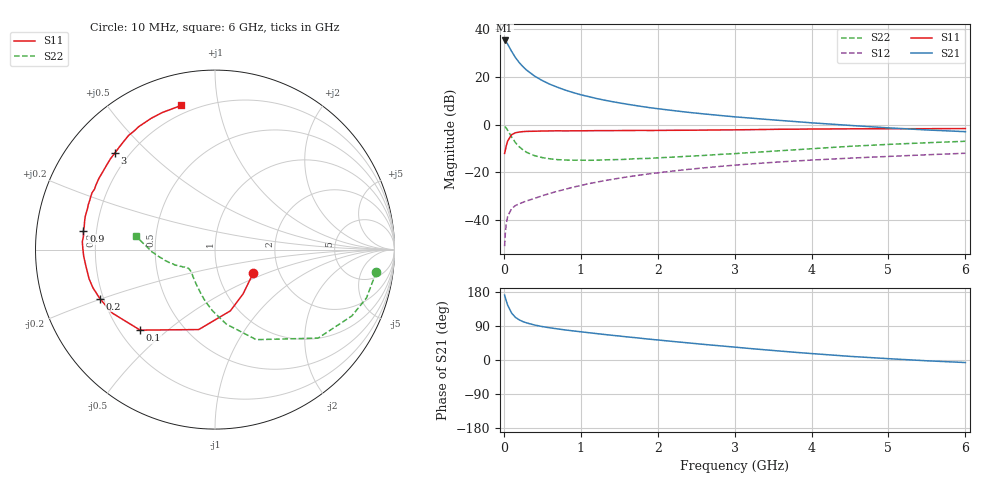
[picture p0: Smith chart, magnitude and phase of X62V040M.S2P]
! SIEMENS Small Signal Semiconductors
! BFP193W
! Si NPN RF Bipolar Junction Transistor in SOT343
! VCE = 2 V  IC = 40 mA
! Common Emitter S-Parameters:  April 1994
# GHz  S  MA  R  50
!  f  S11  S21  S12  S22
! GHz  MAG  ANG  MAG  ANG  MAG  ANG  MAG  ANG
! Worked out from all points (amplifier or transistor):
!   40 points, 10 MHz to 6 GHz, reference 50 ohm
!   highest |S21| = 35.1 dB at 10 MHz (marker M1)
!   |S21| within 3 dB of that: start of sweep to 74.51 MHz
!   unconditionally stable (mu >= 1): 607.5 MHz to 3.992 GHz
!   at 200 MHz: K = 0.55, MSG = 29.5 dB, |S12| = -33.1 dB
!   at 1.5 GHz: K = 1.14, MAG = 13.4 dB, |S12| = -22.4 dB
!   at 6 GHz: K = 0.94, MSG = 4.5 dB, |S12| = -12.0 dB
!   S11 on the Smith chart (normalised r, x): 10 MHz: 1.47, -0.41; 100 MHz: 0.28, -0.41; 200 MHz: 0.19, -0.20; 900 MHz: 0.15, +0.07; 3 GHz: 0.15, +0.40; 6 GHz: 0.16, +0.78
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0.01  0.2499 -31.6  56.79 171.3  0.0029 82.3  0.9072 -7.9
0.02  0.2925 -57.7  55.65 164.2  0.0056 71.2  0.886 -17.7
0.03  0.3518 -75.9  53.4 157.0  0.008 71.4  0.8469 -25.9
0.05  0.4546 -101.5  47.42 144.4  0.0122 61.5  0.7574 -40.6
0.1  0.6125 -132.9  33.87 124.1  0.0175 48.7  0.5519 -65.4
0.15  0.6728 -148.3  25.07 112.6  0.0204 44.2  0.4208 -81.2
0.2  0.6974 -157.0  19.58 105.9  0.0222 43.5  0.3433 -92.0
0.25  0.7127 -162.7  16.06 101.1  0.0239 44.1  0.2959 -100.1
0.3  0.7203 -167.0  13.49 97.7  0.0256 45.2  0.2613 -107.0
0.4  0.7252 -172.8  10.25 92.3  0.0288 48.6  0.224 -116.8
0.5  0.7323 -177.0  8.271 88.2  0.0327 52.1  0.2044 -124.2
0.6  0.7364 179.6  6.911 84.9  0.0366 54.5  0.1924 -130.0
0.8  0.7366 174.2  5.222 79.3  0.0447 58.2  0.1817 -136.8
0.9  0.7405 171.9  4.652 76.8  0.0493 59.3  0.1804 -139.4
1.1  0.7434 167.8  3.833 72.1  0.0582 60.5  0.1795 -143.2
1.6  0.7499 158.4  2.661 61.0  0.0806 60.8  0.1886 -148.0
2.2  0.7588 148.5  1.958 48.9  0.1073 58.3  0.2092 -153.5
3  0.7751 136.0  1.449 34.0  0.142 53.1  0.2471 -161.1
3.2  0.7818 132.9  1.366 30.3  0.1502 51.6  0.2598 -163.1
4.5  0.8133 115.9  0.959 9.6  0.199 41.9  0.3515 -178.0
5.5  0.8194 107.3  0.771 -2.1  0.234 35.1  0.4171 173.3
6  0.8247 103.2  0.71 -6.7  0.2518 32.1  0.4476 170.0
